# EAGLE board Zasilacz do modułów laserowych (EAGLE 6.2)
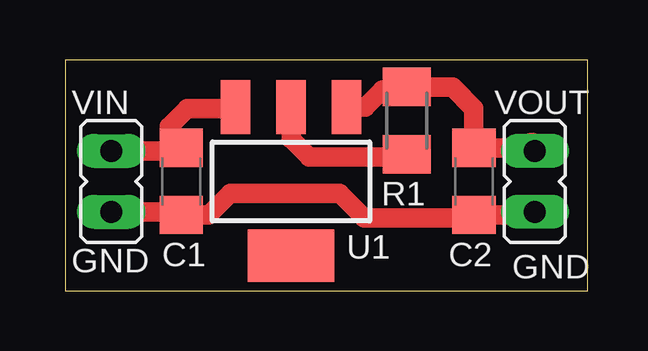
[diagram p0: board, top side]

Size 21.77 x 9.64 mm. Coordinates in mm from the lower left corner, seen from the top.
Outline: 0,0 21.77,0 21.77,9.64 0,9.64 0,0
Copper layers (1*16): Top 0.035mm / dielectric 1.5mm / Bottom 0.035mm
Design rules: minimum track width 10mil, minimum drill 24mil, track to track 8mil, track to pad 8mil, pad to pad 8mil, via to via 8mil, smd to smd 8mil, copper to edge 40mil, drill to drill 8mil, minimum pad ring 10mil, minimum via ring 8mil, stop-mask expansion 4mil, vias tented up to drill 0mil, thermal gap 10mil

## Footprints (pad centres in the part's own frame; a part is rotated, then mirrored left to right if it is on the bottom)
C1206 = smd 1.6 x 1.8: 1 -1.4,0; 2 1.4,0
M1206 = smd 1.6 x 2: 1 -1.4,0; 2 1.4,0
SOT223 = smd 1.219 x 2.235: 1 -2.311,-3.099; 2 0,-3.099; 3 2.311,-3.099 | smd 3.6 x 2.2: 4 0,3.099
JP1 = drill 0.914 long: 1 0,-1.27; 2 0,1.27

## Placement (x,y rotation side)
C1  100nF  [C1206]  4.83,4.57 90 top
C2  100nF  [C1206]  17.02,4.57 90 top
R1  56  [M1206]  14.22,7.11 90 top
U1  LM317  [SOT223]  9.4,4.57 180 top
VIN  [JP1]  1.91,4.57 0 top
VOUT  [JP1]  19.56,4.57 180 top

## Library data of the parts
C1 C2 R1 = rcl
U1 = moja
VIN VOUT = jumper

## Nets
N$1: R1.1 U1.2
N$2: C2.2 R1.2 U1.1 VOUT.1
N$3: C1.2 U1.3 VIN.2
N$4: C1.1 C2.1 VIN.1 VOUT.2

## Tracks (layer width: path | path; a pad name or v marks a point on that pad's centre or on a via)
N$1
  Top 0.813: U1.2 9.4,6.35 10.16,5.59 14.35,5.59 R1.1
N$2
  Top 0.813: U1.1 12.5,7.67 13.21,8.38 14.35,8.38 R1.2 16.13,8.51 17.02,7.62 C2.2 19.43,5.97
  Top 1.27: 19.43,5.97 VOUT.1
N$3
  Top 0.813: VIN.2 4.19,5.84 C1.2 4.32,6.86 5.08,7.62 7.04,7.62 U1.3
N$4
  Top 0.813: VIN.1 4.19,3.3 C1.1 5.97,3.17 6.86,4.06 11.43,4.06 12.45,3.05 16.89,3.05 C2.1 19.43,3.17 VOUT.2

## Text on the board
tNames: GND | GND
